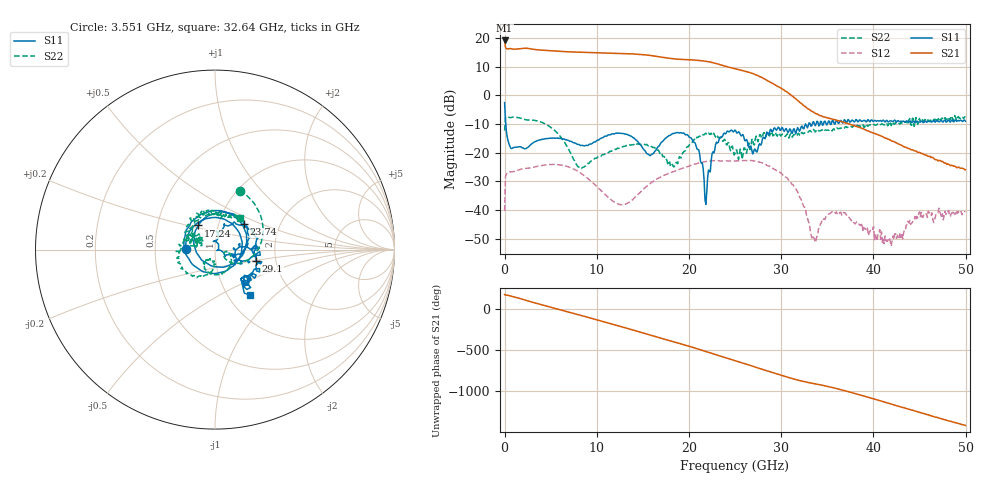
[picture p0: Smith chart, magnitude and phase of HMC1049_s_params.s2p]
!Agilent Technologies,E8361A,US43140893,A.06.04.32
!Agilent HMC1049: A.06.04.32
!Date: Wednesday, November 18, 2012 13:50:33
!Correction: S11(Full 2 Port(1,2)) S21(Full 2 Port(1,2)) S12(Full 2 Port(1,2)) S22(Full 2 Port(1,2))
!S2P File: Measurements: S11, S21, S12, S22:
# GHz S  dB  R 50
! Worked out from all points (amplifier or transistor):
!   523 points, 10 MHz to 49.97 GHz, reference 50 ohm
!   highest |S21| = 19.1 dB at 10 MHz (marker M1)
!   |S21| within 3 dB of that: 1.35 GHz to 2.953 GHz (1.603 GHz wide, 74.5 % of centre)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
!   unconditionally stable (mu >= 1): start of sweep to end of sweep
!   at 8.336 GHz: K = 2.14, MAG = 15.1 dB, |S12| = -27.3 dB
!   at 24.99 GHz: K = 2.35, MAG = 9.6 dB, |S12| = -23.0 dB
!   at 49.97 GHz: K = 759.60, MAG = -24.5 dB, |S12| = -40.6 dB
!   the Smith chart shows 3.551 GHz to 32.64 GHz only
!   S11 on the Smith chart (normalised r, x): 3.551 GHz: 0.72, +0.01; 17.24 GHz: 0.80, +0.22; 23.74 GHz: 1.32, +0.39; 29.1 GHz: 1.58, -0.22; 32.64 GHz: 1.26, -0.71
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0.01  -2.54 -9.5  19.14 175.6  -40.30 78.8  -12.31 -174.1
2.2111  -18.69 -134.1  16.42 109.9  -25.54 -55.6  -8.49 108.8
3.5509  -15.82 178.2  15.89 66.2  -24.81 -96.4  -8.95 67.2
4.795  -15.04 127.2  15.59 28.2  -24.19 -140.3  -10.67 23.6
5.8477  -15.01 83.8  15.38 -4.0  -24.22 179.3  -13.62 -11.6
8.3359  -17.51 -56.6  15.00 -79.4  -27.32 77.4  -25.61 -20.8
9.8671  -16.23 -160.4  14.86 -126.6  -31.42 17.0  -21.98 -10.8
11.7811  -13.45 107.7  14.65 173.5  -37.02 -61.4  -19.15 -33.8
14.2693  -15.68 -2.5  14.39 93.4  -35.19 162.5  -17.27 -77.8
16.6618  -17.93 159.2  13.49 14.3  -28.96 56.1  -19.07 -125.3
17.236  -15.74 124.4  13.19 -4.0  -28.00 33.9  -21.34 -132.8
18.7672  -12.98 59.1  12.59 -52.0  -26.15 -20.8  -23.90 -92.9
20.107  -14.70 9.1  12.39 -95.2  -24.55 -66.6  -16.93 -104.8
22.021  -28.83 56.8  11.77 -162.7  -23.00 -136.2  -13.61 -157.8
23.7436  -13.40 41.1  10.33 136.5  -22.90 162.0  -15.94 151.2
25.0834  -12.48 3.1  9.20 90.7  -22.95 116.9  -19.18 140.9
26.9974  -19.83 -20.0  7.47 22.0  -22.89 45.5  -17.07 164.2
29.1028  -12.44 -15.8  4.07 -54.0  -25.54 -37.3  -14.16 108.3
32.6437  -9.96 -52.6  -4.00 -165.0  -40.18 -163.2  -12.92 52.0
33.4093  -9.51 -67.7  -5.69 177.4  -48.93 -155.2  -12.23 39.5
41.6395  -9.29 -174.4  -15.39 -65.4  -49.85 -4.1  -10.19 -64.4
49.9654  -9.05 83.7  -25.97 25.9  -40.56 140.7  -7.39 -138.3
